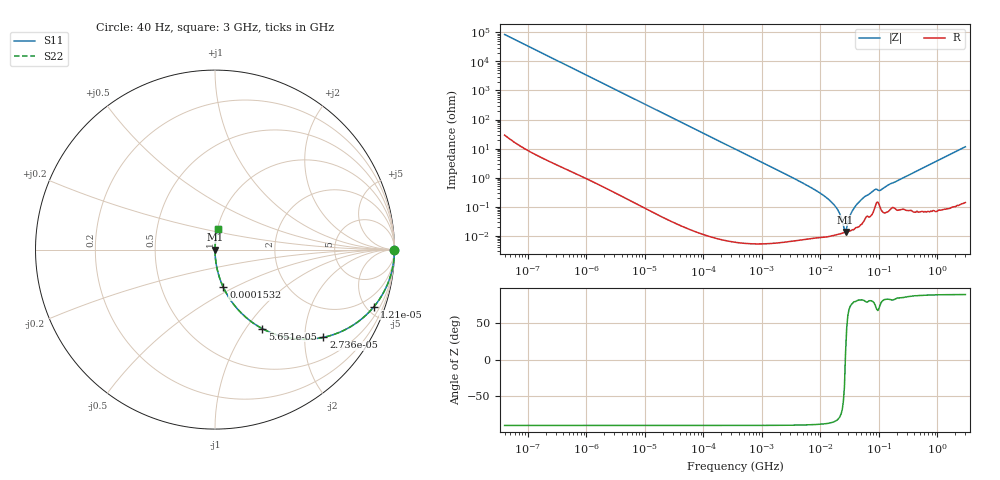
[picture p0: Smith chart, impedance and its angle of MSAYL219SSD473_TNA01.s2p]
! MSAYL219SSD473_TNA01  S-PARAMETER MODEL  ( General Type )
! Model Generated by TAIYO YUDEN Corporation (http://www.ty-top.com)
! Version 2.0
! TAIYO YUDEN Control No. 031016
! Copyright(c) 2003 TAIYO YUDEN CO.,LTD. All Rights Reserved.
! Product Description (link to TY-COMPAS)
! https://ds.yuden.co.jp/TYCOMPAS/or/detail?pn=MSAYL219SSD473KTNA01&u=M
! Products Name : Multilayer Ceramic Capacitors
! Characteristics :
!  Capacitance : 0.047 uF , Rated Voltage : 10V
!  Case Size : 2.0 x 1.25 / 0.079 x 0.049 [mm/inch] , Thickness : 0.85 / 0.033 [mm/inch]
!  (Conditions: Temperature = 25 degC , DC Bias Current/Voltage = 0A / 0V)
! External Node Assignments :
!  1  o---| |---o  2
! GND o---------o GND
! Frequency Range : 40Hz  -  3GHz  [ 401 STEP ]
# MHz S RI R 50
! Freq[MHz].  S11 Real  S11 Imag  S21 Real  S21 Imag  S12 Real  S12 Imag  S22 Real  S22 Imag
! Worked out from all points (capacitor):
!   401 points, 40 Hz to 3 GHz, reference 50 ohm
!   read as one part in series: C = 47.1 nF near 44 Hz
!   lowest |Z| = 13.4 mohm at 26.89 MHz (marker M1)
!   series resonance near 26.65 MHz, so ESL is about 760 pH
!   S11 on the Smith chart (normalised r, x): 40 Hz: open; 12.1 kHz: 1.00, -5.59; 27.36 kHz: 1.00, -2.47; 56.51 kHz: 1.00, -1.20; 153.2 kHz: 1.00, -0.44; 3 GHz: 1.00, +0.23
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4e-05  1 -0.00118  1.8e-06 0.00118  1.8e-06 0.00118  1 -0.00118
0.000834  0.9994 -0.0246  0.000614 0.0246  0.000614 0.0246  0.9994 -0.0246
0.003895  0.9869 -0.1136  0.0131 0.1136  0.0131 0.1136  0.9869 -0.1136
0.012098  0.8865 -0.3171  0.1135 0.3171  0.1135 0.3171  0.8865 -0.3171
0.017386  0.7909 -0.4065  0.2091 0.4065  0.2091 0.4065  0.7909 -0.4065
0.027358  0.6045 -0.4888  0.3955 0.4888  0.3955 0.4888  0.6045 -0.4888
0.056505  0.2639 -0.4406  0.7361 0.4406  0.7361 0.4406  0.2639 -0.4406
0.153184  0.0466 -0.2105  0.9534 0.2105  0.9534 0.2105  0.0466 -0.2105
0.362475  0.00869 -0.0925  0.9913 0.0925  0.9913 0.0925  0.00869 -0.0925
7.222098  9.98e-05 -0.00433  0.9999 0.00433  0.9999 0.00433  9.98e-05 -0.00433
11.89125  9.48e-05 -0.00226  0.9999 0.00226  0.9999 0.00226  9.48e-05 -0.00226
17.08948  0.000105 -0.00116  0.9999 0.00116  0.9999 0.00116  0.000105 -0.00116
20.48705  0.000114 -0.000671  0.9999 0.000671  0.9999 0.000671  0.000114 -0.000671
24.56009  0.000125 -0.000202  0.9999 0.000202  0.9999 0.000202  0.000125 -0.000202
26.8909  0.000132 2.49e-05  0.9999 -2.49e-05  0.9999 -2.49e-05  0.000132 2.49e-05
28.13798  0.000136 0.000132  0.9999 -0.000132  0.9999 -0.000132  0.000136 0.000132
35.29647  0.000162 0.000715  0.9998 -0.000715  0.9998 -0.000715  0.000162 0.000715
48.47801  0.00024 0.00164  0.9998 -0.00164  0.9998 -0.00164  0.00024 0.00164
83.52119  0.000857 0.00367  0.9991 -0.00367  0.9991 -0.00367  0.000857 0.00367
109.6283  0.000768 0.00377  0.9992 -0.00377  0.9992 -0.00377  0.000768 0.00377
150.5692  0.000773 0.00582  0.9992 -0.00582  0.9992 -0.00582  0.000773 0.00582
3000  0.0145 0.1135  0.9855 -0.1135  0.9855 -0.1135  0.0145 0.1135
